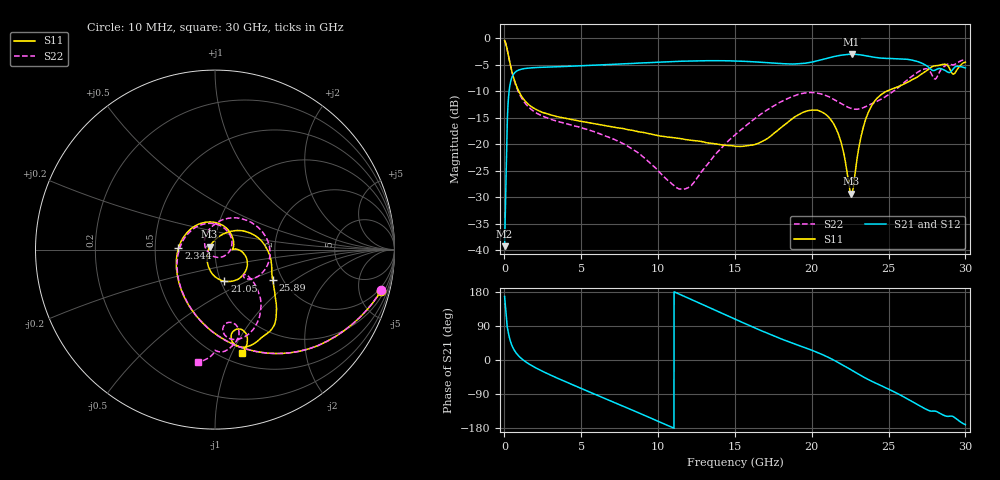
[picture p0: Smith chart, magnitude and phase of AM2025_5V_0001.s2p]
!Keysight Technologies,N5245B,MY58422270,A.16.20.02
!Date: Tuesday, July 14, 2026 00:50:50
!Correction: S11(C  2-Port  )
!S21(C  2-Port  )
!S12(C  2-Port  )
!S22(C  2-Port  )
!S2P File: Measurements: S11, S21, S12, S22:
# Hz S  dB  R 50
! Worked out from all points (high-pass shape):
!   3201 points, 10 MHz to 30 GHz, reference 50 ohm
!   highest |S21| = -3.01 dB at 22.6 GHz (marker M1); lowest = -39.2 dB at 10 MHz (marker M2)
!   |S21| within 3 dB of the highest: 910.8 MHz to 27.82 GHz (26.91 GHz wide, 187 % of centre); 29.14 GHz to end of sweep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
!   lowest |S11| = -29.3 dB at 22.58 GHz (marker M3), VSWR 1.07, Z = 47.1 + j1.54 ohm
!   |S11| at or under -10 dB: 933.5 MHz to 24.86 GHz (23.92 GHz wide, 186 % of centre)
!   |S22| runs from -28.5 to -0.4 dB; largest |S21 - S12| = 0.024
!   S11 on the Smith chart (normalised r, x): 10 MHz: 1.56, -7.81; 2.344 GHz: 0.66, +0.01; 21.05 GHz: 1.04, -0.38; 25.89 GHz: 1.78, -0.69; 30 GHz: 0.61, -1.09
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1e7  -0.42 -14.0  -39.21 167.8  -32.84 124.4  -0.41 -13.7
2.536688e8  -3.20 -56.7  -11.52 71.8  -11.52 71.7  -3.24 -57.2
4.317344e8  -5.63 -81.1  -7.85 44.2  -7.85 44.1  -5.70 -81.9
9.84675e8  -10.29 -125.7  -5.93 8.3  -5.93 8.3  -10.58 -128.3
2.343597e9  -13.82 178.1  -5.48 -27.1  -5.47 -27.1  -14.50 168.2
5.014581e9  -15.69 116.0  -5.19 -75.4  -5.18 -75.5  -16.88 89.6
7.441897e9  -16.92 74.1  -4.86 -117.1  -4.86 -117.2  -19.47 28.3
1.000979e10  -18.35 39.2  -4.51 -161.8  -4.51 -161.8  -24.97 -45.8
1.189354e10  -19.13 19.7  -4.30 164.5  -4.29 164.5  -28.27 -145.3
1.5005e10  -20.36 0.2  -4.28 108.0  -4.27 107.8  -18.20 102.0
1.773222e10  -17.47 -0.7  -4.72 60.2  -4.72 60.1  -12.40 43.0
2.000958e10  -13.56 -40.4  -4.49 25.8  -4.48 25.7  -10.23 -9.2
2.104986e10  -14.71 -73.4  -3.73 7.6  -3.74 7.5  -10.94 -31.3
2.18371e10  -18.97 -106.1  -3.23 -9.2  -3.22 -9.2  -12.20 -41.8
2.257748e10  -29.33 151.4  -3.01 -26.4  -3.02 -26.5  -13.24 -43.3
2.259622e10  -29.29 145.9  -3.01 -26.9  -3.02 -26.9  -13.26 -43.2
2.357089e10  -14.78 35.3  -3.31 -49.3  -3.31 -49.3  -12.80 -38.6
2.500479e10  -9.81 -13.6  -3.81 -77.0  -3.80 -77.1  -10.62 -41.0
2.588575e10  -8.78 -27.7  -3.88 -95.0  -3.88 -95.2  -8.66 -46.8
2.73009e10  -6.45 -43.9  -4.88 -127.1  -4.88 -127.3  -5.81 -71.0
2.899721e10  -5.86 -79.7  -6.43 -148.1  -6.41 -148.3  -4.90 -88.1
3e10  -4.51 -75.3  -5.59 -170.5  -5.58 -170.8  -3.96 -98.5
